| TEXAS INSTRUMENTS INCORPORATED
| Standard Linear and Logic Group
| IBIS Model of SN74LVC821A
| 10-Bit Bus-Interface Flip-Flop with 3-State Outputs
| This file contains package information for the following:
|  TSSOP 24-pin (PW) package as [Component] LVC821A_PW
|  SSOP 24-pin (DB) package as [Component] LVC821A_DB
|  TVSOP 24-pin (DGV) package as [Component] LVC821A_DGV
|  SOIC 24-pin (DW) package as [Component] LVC821A_DW
|  SOP 24-pin (NS) package as [Component] LVC821A_NS
| This device can be powered at the following Vccs:
|  1.8 volt Vcc
|  2.5 volt Vcc
|  3.3 volt Vcc
| This file provides unique models under the [Model Selector] for each Vcc.
| For operation at a specific Vcc, select the appropriate model after each
| [Model Selector] keyword.
[IBIS Ver]   3.2
[Comment char]  |_char
[File Name]   sn74lvc821a.ibs
[File Rev]   1.1 | a
[Date]   August 22, 2007
[Source]   Data created from TI-SPICE simulations at TI-SLL.
[Notes]   The following is an IBIS list for the LVC821A.
   Please contact sllibis@ti.com with questions and
   comments concerning SLL IBIS models.
   This IBIS model is created from a BA (back annotated netlist)
   - FILE REV HISTORY
   - 1.1 Release IBIS file on 08/23/07
   - Power-clamp data has been deleted since there is no
   power-clamp diode in the device.
   - Due to the fact that the device is 5-V input/output
   tolerant, the pullup data has some non-monotonic warnings.
   - End point warning due to AC and DC mismatch.
[Disclaimer] Property of Texas Instruments Incorporated.  Unauthorized
   reproduction and/or distribution is strictly prohibited.
   This product is protected under copyright law.
   Created  2005, (C) Copyright  2005, Texas Instruments
   Incorporated, All Rights Reserved
   UNLESS THERE IS A SIGNED, WRITTEN AGREEMENT TO THE
   CONTRARY, TEXAS INSTRUMENTS (TI) IS PROVIDING THE IBIS
   MODELS  AND WITHOUT ANY WARRANTY, EXPRESSED OR
   IMPLIED.  TI assumes no liability for:
   1) the accuracy of the IBIS models provided to your
   company;
   2) the proper functioning of these IBIS Models in your
   design or for any resulting applications; or
   3) infringement of patents, copyrights or intellectual
   property rights resulting from your use of these IBIS
   models.
   TI provides IBIS Models as a service to our customers.
   You and your company shall not distribute, sell or give
   these models to anyone else without prior written
   permission from TI.
   TI reserves the right to make changes to our products or
   to discontinue any semiconductor product or service
   without notice, and advises our customers to obtain the
   latest version of relevant information to verify, before
   placing orders, that the information being relied on is
   current.
   Please be aware that your receipt and use of the IBIS
   information provided shall serve as acceptance of these
   terms and conditions.  If you do not accept these terms,
   you should return or destroy the IBIS models and any
   other accompanying information immediately.
| Component LVC821A_PW 24-pin TSSOP
[Component]   LVC821A_PW
[Manufacturer]   Texas Instruments, Inc.
[Package]
|   typ   min   max
R_pkg   3.900e-02   3.000e-02   4.600e-02
L_pkg   2.685e-09   2.367e-09   3.177e-09
C_pkg   3.200e-13   2.520e-13   4.340e-13
[Pin]   signal_name   model_name   R_pin   L_pin   C_pin
1   NOE   LVC821A_NOE   3.700e-02   3.153e-09   4.340e-13
2   1D   LVC821A_IN   3.400e-02   2.629e-09   3.410e-13
3   2D   LVC821A_IN   3.200e-02   2.860e-09   3.470e-13
4   3D   LVC821A_IN   4.200e-02   2.741e-09   2.900e-13
5   4D   LVC821A_IN   4.600e-02   2.600e-09   2.620e-13
6   5D   LVC821A_IN   4.300e-02   2.414e-09   2.660e-13
7   6D   LVC821A_IN   4.200e-02   2.367e-09   2.620e-13
8   7D   LVC821A_IN   4.400e-02   2.461e-09   2.520e-13
9   8D   LVC821A_IN   4.200e-02   2.543e-09   2.740e-13
10   9D   LVC821A_IN   3.000e-02   2.616e-09   3.320e-13
11   10D   LVC821A_IN   3.700e-02   2.670e-09   3.460e-13
12   GND   GND   3.900e-02   3.177e-09   4.330e-13
13   CLK   LVC821A_CLK   3.700e-02   3.111e-09   4.310e-13
14   10Q   LVC821A_OUT   3.700e-02   2.656e-09   3.450e-13
15   9Q   LVC821A_OUT   3.100e-02   2.739e-09   3.400e-13
16   8Q   LVC821A_OUT   4.200e-02   2.649e-09   2.820e-13
17   7Q   LVC821A_OUT   4.600e-02   2.532e-09   2.570e-13
18   6Q   LVC821A_OUT   4.400e-02   2.425e-09   2.660e-13
19   5Q   LVC821A_OUT   4.400e-02   2.425e-09   2.660e-13
20   4Q   LVC821A_OUT   4.600e-02   2.532e-09   2.570e-13
21   3Q   LVC821A_OUT   4.200e-02   2.648e-09   2.820e-13
22   2Q   LVC821A_OUT   3.100e-02   2.738e-09   3.390e-13
23   1Q   LVC821A_OUT   3.600e-02   2.653e-09   3.440e-13
24   VCC   POWER   3.700e-02   3.110e-09   4.310e-13
| Component LVC821A_DB 24-pin SSOP
[Component]   LVC821A_DB
[Manufacturer]   Texas Instruments, Inc.
[Package]
|   typ   min   max
R_pkg   4.500e-02   4.000e-02   4.900e-02
L_pkg   3.668e-09   3.226e-09   4.415e-09
C_pkg   4.160e-13   3.490e-13   5.070e-13
[Pin]   signal_name   model_name   R_pin   L_pin   C_pin
1   NOE   LVC821A_NOE   4.200e-02   4.299e-09   5.030e-13
2   1D   LVC821A_IN   4.000e-02   3.960e-09   4.990e-13
3   2D   LVC821A_IN   4.200e-02   3.775e-09   4.170e-13
4   3D   LVC821A_IN   4.700e-02   3.487e-09   3.690e-13
5   4D   LVC821A_IN   4.600e-02   3.347e-09   3.520e-13
6   5D   LVC821A_IN   4.900e-02   3.352e-09   3.710e-13
7   6D   LVC821A_IN   4.600e-02   3.226e-09   3.630e-13
8   7D   LVC821A_IN   4.700e-02   3.289e-09   3.490e-13
9   8D   LVC821A_IN   4.700e-02   3.347e-09   3.610e-13
10   9D   LVC821A_IN   4.100e-02   3.576e-09   4.090e-13
11   10D   LVC821A_IN   4.100e-02   3.995e-09   5.030e-13
12   GND   GND   4.500e-02   4.415e-09   5.070e-13
13   CLK   LVC821A_CLK   4.300e-02   4.337e-09   5.060e-13
14   10Q   LVC821A_OUT   4.200e-02   4.003e-09   5.040e-13
15   9Q   LVC821A_OUT   4.100e-02   3.686e-09   4.100e-13
16   8Q   LVC821A_OUT   4.800e-02   3.355e-09   3.490e-13
17   7Q   LVC821A_OUT   4.700e-02   3.301e-09   3.530e-13
18   6Q   LVC821A_OUT   4.800e-02   3.268e-09   3.660e-13
19   5Q   LVC821A_OUT   4.800e-02   3.269e-09   3.660e-13
20   4Q   LVC821A_OUT   4.700e-02   3.314e-09   3.490e-13
21   3Q   LVC821A_OUT   4.800e-02   3.399e-09   3.550e-13
22   2Q   LVC821A_OUT   4.100e-02   3.688e-09   4.120e-13
23   1Q   LVC821A_OUT   4.200e-02   4.003e-09   5.040e-13
24   VCC   POWER   4.300e-02   4.347e-09   5.050e-13
| Component LVC821A_DGV 24-pin TVSOP
[Component]   LVC821A_DGV
[Manufacturer]   Texas Instruments, Inc.
[Package]
|   typ   min   max
R_pkg   4.300e-02   3.900e-02   4.700e-02
L_pkg   2.601e-09   2.312e-09   3.626e-09
C_pkg   3.580e-13   2.770e-13   5.950e-13
[Pin]   signal_name   model_name   R_pin   L_pin   C_pin
1   NOE   LVC821A_NOE   4.300e-02   3.625e-09   5.950e-13
2   1D   LVC821A_IN   4.000e-02   2.656e-09   4.020e-13
3   2D   LVC821A_IN   3.900e-02   2.338e-09   3.080e-13
4   3D   LVC821A_IN   4.600e-02   2.354e-09   2.770e-13
5   4D   LVC821A_IN   4.500e-02   2.312e-09   2.850e-13
6   5D   LVC821A_IN   4.700e-02   2.318e-09   2.820e-13
7   6D   LVC821A_IN   4.700e-02   2.318e-09   2.820e-13
8   7D   LVC821A_IN   4.500e-02   2.312e-09   2.850e-13
9   8D   LVC821A_IN   4.600e-02   2.353e-09   2.780e-13
10   9D   LVC821A_IN   3.900e-02   2.338e-09   3.080e-13
11   10D   LVC821A_IN   4.100e-02   2.660e-09   4.020e-13
12   GND   GND   4.300e-02   3.625e-09   5.950e-13
13   CLK   LVC821A_CLK   4.400e-02   3.626e-09   5.940e-13
14   10Q   LVC821A_OUT   4.000e-02   2.658e-09   4.020e-13
15   9Q   LVC821A_OUT   3.900e-02   2.343e-09   3.110e-13
16   8Q   LVC821A_OUT   4.600e-02   2.353e-09   2.780e-13
17   7Q   LVC821A_OUT   4.500e-02   2.312e-09   2.850e-13
18   6Q   LVC821A_OUT   4.700e-02   2.319e-09   2.820e-13
19   5Q   LVC821A_OUT   4.700e-02   2.319e-09   2.820e-13
20   4Q   LVC821A_OUT   4.500e-02   2.312e-09   2.850e-13
21   3Q   LVC821A_OUT   4.600e-02   2.353e-09   2.780e-13
22   2Q   LVC821A_OUT   3.900e-02   2.337e-09   3.080e-13
23   1Q   LVC821A_OUT   4.000e-02   2.658e-09   4.020e-13
24   VCC   POWER   4.400e-02   3.626e-09   5.950e-13
| Component LVC821A_DW 24-pin SOIC
[Component]   LVC821A_DW
[Manufacturer]   Texas Instruments, Inc.
[Package]
|   typ   min   max
R_pkg   3.700e-02   3.000e-02   4.700e-02
L_pkg   5.146e-09   3.993e-09   6.885e-09
C_pkg   7.580e-13   5.120e-13   1.067e-12
[Pin]   signal_name   model_name   R_pin   L_pin   C_pin
1   NOE   LVC821A_NOE   3.900e-02   6.885e-09   1.067e-12
2   1D   LVC821A_IN   4.200e-02   5.950e-09   9.580e-13
3   2D   LVC821A_IN   4.700e-02   5.317e-09   7.910e-13
4   3D   LVC821A_IN   3.100e-02   4.651e-09   6.110e-13
5   4D   LVC821A_IN   3.000e-02   3.993e-09   5.120e-13
6   5D   LVC821A_IN   3.000e-02   4.083e-09   6.110e-13
7   6D   LVC821A_IN   3.000e-02   4.083e-09   6.110e-13
8   7D   LVC821A_IN   3.000e-02   3.993e-09   5.120e-13
9   8D   LVC821A_IN   3.100e-02   4.652e-09   6.110e-13
10   9D   LVC821A_IN   4.700e-02   5.317e-09   7.910e-13
11   10D   LVC821A_IN   4.200e-02   5.950e-09   9.590e-13
12   GND   GND   3.900e-02   6.885e-09   1.067e-12
13   CLK   LVC821A_CLK   3.900e-02   6.885e-09   1.067e-12
14   10Q   LVC821A_OUT   4.200e-02   5.950e-09   9.590e-13
15   9Q   LVC821A_OUT   4.700e-02   5.317e-09   7.910e-13
16   8Q   LVC821A_OUT   3.100e-02   4.652e-09   6.110e-13
17   7Q   LVC821A_OUT   3.000e-02   3.993e-09   5.120e-13
18   6Q   LVC821A_OUT   3.000e-02   4.083e-09   6.100e-13
19   5Q   LVC821A_OUT   3.000e-02   4.083e-09   6.100e-13
20   4Q   LVC821A_OUT   3.000e-02   3.993e-09   5.120e-13
21   3Q   LVC821A_OUT   3.100e-02   4.651e-09   6.110e-13
22   2Q   LVC821A_OUT   4.700e-02   5.317e-09   7.910e-13
23   1Q   LVC821A_OUT   4.200e-02   5.950e-09   9.580e-13
24   VCC   POWER   3.900e-02   6.885e-09   1.067e-12
| Component LVC821A_NS 24-pin SOP
[Component]   LVC821A_NS
[Manufacturer]   Texas Instruments, Inc.
[Package]
|   typ   min   max
R_pkg   4.400e-02   3.800e-02   4.800e-02
L_pkg   3.840e-09   2.545e-09   5.234e-09
C_pkg   5.860e-13   2.740e-13   7.970e-13
[Pin]   signal_name   model_name   R_pin   L_pin   C_pin
1   NOE   LVC821A_NOE   4.100e-02   5.146e-09   7.650e-13
2   1D   LVC821A_IN   4.100e-02   4.357e-09   7.490e-13
3   2D   LVC821A_IN   4.000e-02   3.923e-09   6.330e-13
4   3D   LVC821A_IN   4.400e-02   3.412e-09   5.370e-13
5   4D   LVC821A_IN   4.500e-02   3.036e-09   3.970e-13
6   5D   LVC821A_IN   4.500e-02   2.845e-09   4.150e-13
7   6D   LVC821A_IN   4.400e-02   2.843e-09   4.150e-13
8   7D   LVC821A_IN   4.500e-02   3.065e-09   3.990e-13
9   8D   LVC821A_IN   4.500e-02   3.529e-09   5.440e-13
10   9D   LVC821A_IN   4.100e-02   4.013e-09   6.390e-13
11   10D   LVC821A_IN   4.100e-02   4.358e-09   7.460e-13
12   GND   GND   4.400e-02   5.234e-09   7.670e-13
13   CLK   LVC821A_CLK   3.900e-02   5.181e-09   7.650e-13
14   10Q   LVC821A_OUT   4.800e-02   4.582e-09   7.640e-13
15   9Q   LVC821A_OUT   4.100e-02   4.163e-09   6.550e-13
16   8Q   LVC821A_OUT   4.600e-02   3.613e-09   5.490e-13
17   7Q   LVC821A_OUT   4.700e-02   3.163e-09   4.060e-13
18   6Q   LVC821A_OUT   4.700e-02   2.963e-09   4.220e-13
19   5Q   LVC821A_OUT   4.700e-02   2.919e-09   4.190e-13
20   4Q   LVC821A_OUT   4.800e-02   3.087e-09   4.870e-13
21   3Q   LVC821A_OUT   4.600e-02   4.513e-09   7.600e-13
22   2Q   LVC821A_OUT   4.200e-02   4.505e-09   7.670e-13
23   1Q   LVC821A_OUT   4.200e-02   5.163e-09   7.970e-13
24   VCC   POWER   3.800e-02   2.545e-09   2.740e-13
| Model LVC821A_NOE
[Model Selector]   LVC821A_NOE
LVC821A_NOE_18   1.8 volt Vcc
LVC821A_NOE_25   2.5 volt Vcc
LVC821A_NOE_33   3.3 volt Vcc
| Model LVC821A_CLK
[Model Selector]   LVC821A_CLK
LVC821A_CLK_18   1.8 volt Vcc
LVC821A_CLK_25   2.5 volt Vcc
LVC821A_CLK_33   3.3 volt Vcc
| Model LVC821A_IN
[Model Selector]   LVC821A_IN
LVC821A_IN_18   1.8 volt Vcc
LVC821A_IN_25   2.5 volt Vcc
LVC821A_IN_33   3.3 volt Vcc
| Model LVC821A_OUT
[Model Selector]   LVC821A_OUT
LVC821A_OUT_18   1.8 volt Vcc
LVC821A_OUT_25   2.5 volt Vcc
LVC821A_OUT_33   3.3 volt Vcc
| Models and submodels in the file (12): LVC821A_NOE_18 (Input), LVC821A_NOE_25 (Input), LVC821A_NOE_33 (Input), LVC821A_CLK_18 (Input), LVC821A_CLK_25 (Input), LVC821A_CLK_33 (Input), LVC821A_IN_18 (Input), LVC821A_IN_25 (Input), LVC821A_IN_33 (Input), LVC821A_OUT_18 (3-state), LVC821A_OUT_25 (3-state), LVC821A_OUT_33 (3-state)
